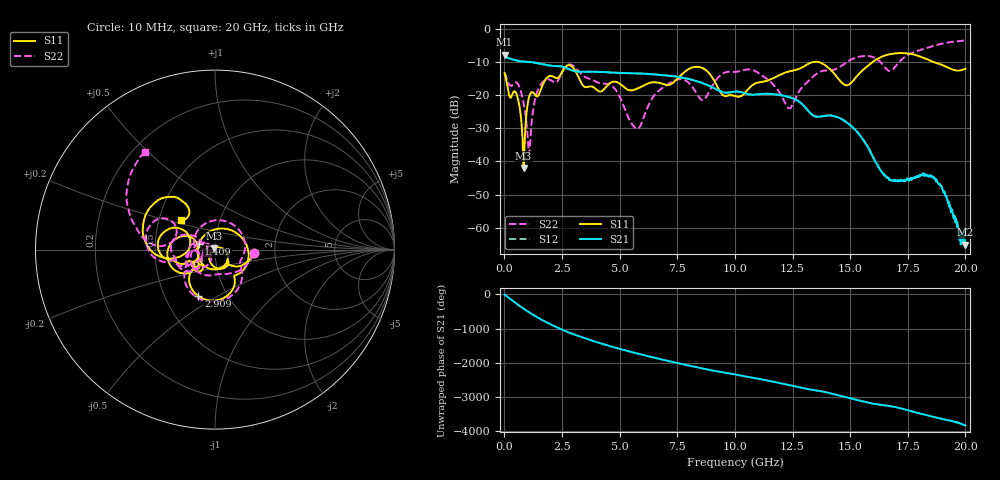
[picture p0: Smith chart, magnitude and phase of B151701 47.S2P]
!  2-Port S-parameters saved by WinCal
! VAR MeasName=S-Parameters (CALIBRATED_DATA) read from VNA (N5244A)
! VAR MeasDate=2015-12-24 19:15:00
! VAR NAME=B151701 47
! VAR FILENAME=B151701 47.S2P
! VAR DATE=2015-12-24 19:15:00
! VAR PHYS_PORTS=1,3
# Hz S DB R 50
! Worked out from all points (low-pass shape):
!   801 points, 10 MHz to 20 GHz, reference 50 ohm
!   highest |S21| = -7.80 dB at 10 MHz (marker M1); lowest = -65.1 dB at 19.98 GHz (marker M2)
!   |S21| within 3 dB of the highest: start of sweep to 1.756 GHz
!   lowest |S11| = -42.0 dB at 834.6 MHz (marker M3), VSWR 1.02, Z = 49.5 + j0.614 ohm
!   |S11| at or under -10 dB: start of sweep to 13.38 GHz; 13.63 GHz to 15.97 GHz (2.343 GHz wide, 15.8 % of centre); 18.63 GHz to end of sweep
!   |S22| runs from -37.7 to -3.5 dB; largest |S21 - S12| = 0.0015
!   S11 on the Smith chart (normalised r, x): 10 MHz: 1.55, -0.07; 1.409 GHz: 0.83, +0.05; 2.909 GHz: 0.73, -0.41; 20 GHz: 0.65, +0.22
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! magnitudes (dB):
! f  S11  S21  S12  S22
! 10 MHz  -13.3  -7.8  -7.8  -13.3
! 559.7 MHz  -20.3  -9.6  -9.6  -16.4
! 834.6 MHz  -42.0  -9.9  -9.9  -22.4
! 1.084 GHz  -20.3  -10.0  -10.0  -37.7
! 1.409 GHz  -20.3  -10.3  -10.3  -19.2
! 2.909 GHz  -11.2  -12.5  -12.5  -10.8
! 3.358 GHz  -16.5  -12.9  -12.9  -13.8
! 4.733 GHz  -15.9  -13.2  -13.2  -17.6
! 5.732 GHz  -18.1  -13.4  -13.4  -30.1
! 6.682 GHz  -16.2  -13.8  -13.8  -18.7
! 7.706 GHz  -13.7  -14.7  -14.7  -15.2
! 8.456 GHz  -11.5  -16.0  -16.0  -20.7
! 10.01 GHz  -20.2  -18.9  -18.9  -13.0
! 11.03 GHz  -16.2  -19.7  -19.7  -13.3
! 12.35 GHz  -12.8  -20.6  -20.6  -24.0
! 13.35 GHz  -10.0  -25.9  -25.9  -14.6
! 14.88 GHz  -17.0  -28.4  -28.3  -9.9
! 15.88 GHz  -10.5  -37.1  -37.0  -8.3
! 16.68 GHz  -7.7  -44.9  -45.4  -12.7
! 18.6 GHz  -9.9  -44.7  -45.1  -5.1
! 19.98 GHz  -12.0  -65.1  -63.9  -3.5
! 20 GHz  -12.0  -64.3  -64.9  -3.5
